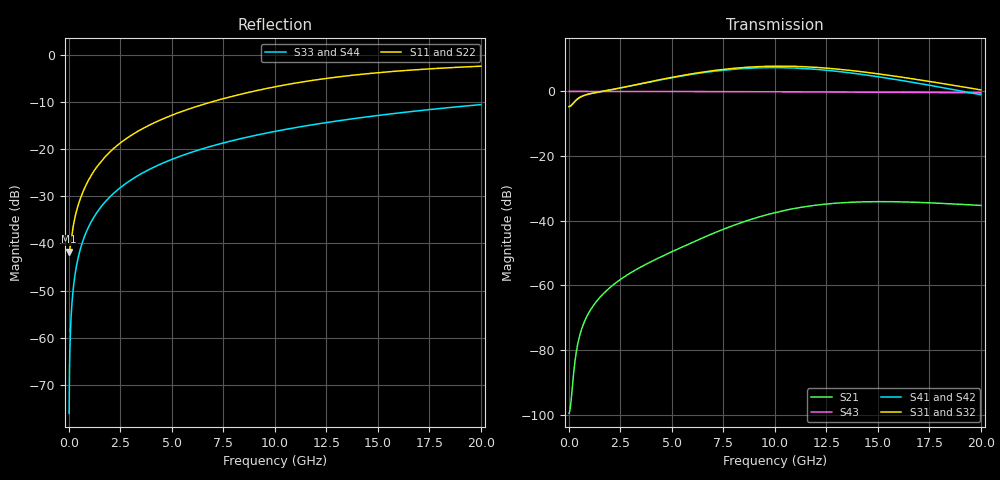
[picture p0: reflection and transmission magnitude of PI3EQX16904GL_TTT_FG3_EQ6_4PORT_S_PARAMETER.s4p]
! NPort=4 DATA=2000 NOISE=0 GROUPDELAY=0 COMPLEX_DATAFORMAT=POLAR
! NumOfBlock=1 NumOfParam=0
! .MODEL Smodel S TSTONEFILE=PI3EQX16904GL_TTT_FG3_EQ6_4PORT_S_PARAMETER.s4p TYPE=S
!  -- The above .MODEL line can be used for the S element in the netlist.
! The s parameter is extracted from the linear redriver, it is not bi-directional; only s(4,1)s(4,2) and s(3,1)s(3,2)
! should be the insertion loss
!Port definition:
!Port1 = input+
!Port2 = input-
!Port3 = output+
!Port4 = output-
# Hz S MA R  50
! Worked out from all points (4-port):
!   2000 points, 10 MHz to 20 GHz, reference 50 ohm
!   strongest paths, dB at 10 MHz, 5.01 GHz, 10.01 GHz, 15.01 GHz, 20 GHz:
!     S31: -4.7, 4.4, 7.8, 5.4, 0.5
!     S32: -4.7, 4.3, 7.7, 5.4, 0.4
!     S41: -4.7, 4.2, 7.4, 4.5, -1.0
!     S42: -4.7, 4.1, 7.3, 4.5, -1.1
!     S43: 0.0, 0.0, -0.1, -0.3, -0.4
!     S21: -99.6, -49.5, -37.5, -34.1, -35.3
!   lowest |S11| = -41.7 dB at 10 MHz (marker M1), VSWR 1.02, Z = 49.2 - j0.0603 ohm
!   |S11| at or under -10 dB: start of sweep to 6.87 GHz
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1e7  0.008182 -175.7  1.05e-05 7.8  0 0.0  0 0.0
     1.05e-05 7.8  0.008182 -175.7  0 0.0  0 0.0
     0.5835 0.7  0.5835 -179.3  0.0001571 -90.0  1 -0.0
     0.5835 -179.3  0.5835 0.7  1 -0.0  0.0001571 -90.0
1.01e9  0.04966 -106.4  0.0003989 111.5  0 0.0  0 0.0
        0.0003988 111.5  0.04966 -106.4  0 0.0  0 0.0
        0.9169 8.3  0.9168 -171.8  0.01586 -90.9  0.9999 -0.9
        0.9164 -173.5  0.9163 6.4  0.9999 -0.9  0.01586 -90.9
5.53e9  0.2545 -104.1  0.003998 102.6  0 0.0  0 0.0
        0.00397 102.9  0.2545 -104.1  0 0.0  0 0.0
        1.772 -32.9  1.749 146.7  0.08651 -95.2  0.996 -5.0
        1.745 137.2  1.722 -43.1  0.996 -5.0  0.08651 -95.2
9.47e9  0.4371 -111.5  0.01212 71.7  0 0.0  0 0.0
        0.01204 72.6  0.437 -111.5  0 0.0  0 0.0
        2.434 -98.2  2.409 81.8  0.147 -98.8  0.9883 -8.5
        2.329 65.3  2.305 -114.8  0.9883 -8.5  0.147 -98.8
1.334e10  0.5975 -121.5  0.01908 23.1  0 0.0  0 0.0
          0.01902 24.3  0.5973 -121.5  0 0.0  0 0.0
          2.164 -167.7  2.144 12.3  0.2047 -102.3  0.9771 -11.8
          1.99 -10.3  1.972 169.6  0.9771 -11.8  0.2047 -102.3
1.612e10  0.6821 -128.4  0.0196 -7.0  0 0.0  0 0.0
          0.01956 -5.5  0.682 -128.4  0 0.0  0 0.0
          1.668 148.4  1.652 -31.7  0.2449 -104.8  0.9671 -14.2
          1.482 -58.4  1.468 121.5  0.9671 -14.2  0.2449 -104.8
2e10  0.7641 -136.3  0.01726 -37.0  0 0.0  0 0.0
      0.01723 -35.2  0.7641 -136.2  0 0.0  0 0.0
      1.055 96.2  1.045 -83.9  0.2986 -108.1  0.9506 -17.4
      0.8884 -115.7  0.8801 64.1  0.9506 -17.4  0.2986 -108.1
